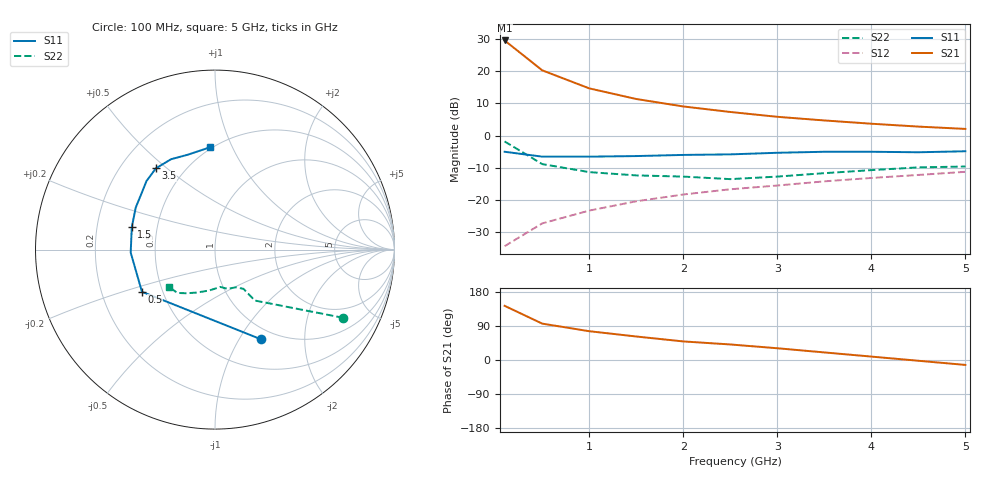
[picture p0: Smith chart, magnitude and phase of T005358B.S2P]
!AT-00535
!S-PARAMETERS at Vce=8V  Ic=20mA.  LAST UPDATED 07-21-92
# ghz s ma r 50
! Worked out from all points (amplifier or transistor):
!   11 points, 100 MHz to 5 GHz, reference 50 ohm
!   highest |S21| = 29.6 dB at 100 MHz (marker M1)
!   |S21| within 3 dB of that: start of sweep to 229.1 MHz
!   unconditionally stable (mu >= 1): 913.6 MHz to 4.422 GHz
!   at 500 MHz: K = 0.82, MSG = 23.8 dB, |S12| = -27.3 dB
!   at 2.5 GHz: K = 1.12, MAG = 9.9 dB, |S12| = -16.7 dB
!   at 5 GHz: K = 0.95, MSG = 6.7 dB, |S12| = -11.3 dB
!   S11 on the Smith chart (normalised r, x): 100 MHz: 0.85, -1.24; 500 MHz: 0.38, -0.23; 1.5 GHz: 0.36, +0.12; 3.5 GHz: 0.35, +0.46; 5 GHz: 0.49, +0.82
0.1  0.56 -63.0  30.24 143.0  0.019 62.0  0.81 -28.0
0.5  0.47 -150.0  10.37 96.0  0.043 54.0  0.36 -52.0
1  0.47 -178.0  5.43 76.0  0.068 56.0  0.27 -54.0
1.5  0.48 165.0  3.71 62.0  0.095 57.0  0.24 -61.0
2  0.5 152.0  2.84 49.0  0.121 53.0  0.23 -72.0
2.5  0.51 145.0  2.33 41.0  0.146 53.0  0.21 -82.0
3  0.54 135.0  1.96 31.0  0.167 50.0  0.23 -98.0
3.5  0.56 126.0  1.72 20.0  0.194 44.0  0.26 -113.0
4  0.56 116.0  1.53 9.0  0.219 40.0  0.29 -123.0
4.5  0.55 106.0  1.38 -2.0  0.244 32.0  0.32 -131.0
5  0.57 93.0  1.27 -13.0  0.273 25.0  0.33 -141.0
